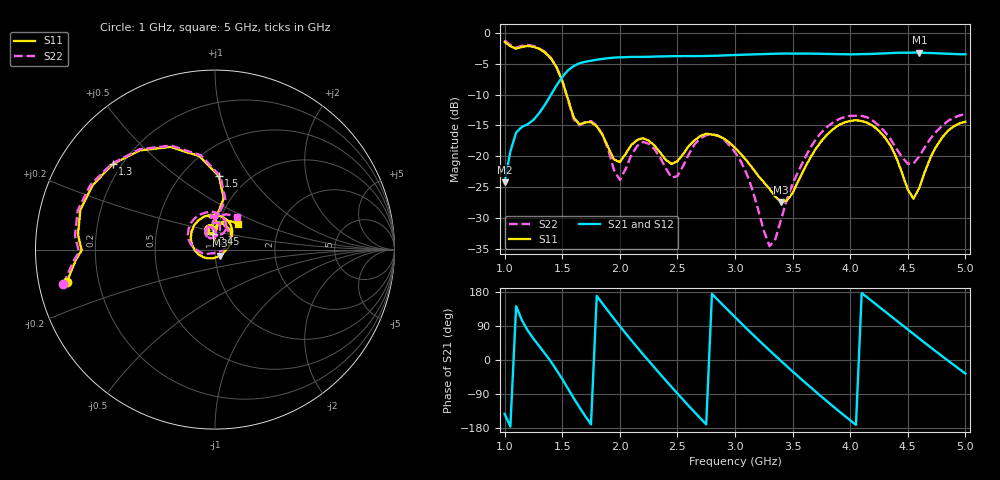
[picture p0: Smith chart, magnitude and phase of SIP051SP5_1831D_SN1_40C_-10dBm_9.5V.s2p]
# GHz  S  dB  R  50
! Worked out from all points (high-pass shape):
!   81 points, 1 GHz to 5 GHz, reference 50 ohm
!   highest |S21| = -3.22 dB at 4.6 GHz (marker M1); lowest = -24.2 dB at 1 GHz (marker M2)
!   |S21| within 3 dB of the highest: 1.544 GHz to end of sweep
!   lowest |S11| = -27.4 dB at 3.4 GHz (marker M3), VSWR 1.09, Z = 52.5 - j3.57 ohm
!   |S11| at or under -10 dB: 1.538 GHz to end of sweep
!   |S22| runs from -34.6 to -1.2 dB; largest |S21 - S12| = 0.0029
!   S11 on the Smith chart (normalised r, x): 1 GHz: 0.09, -0.11; 1.3 GHz: 0.17, +0.35; 1.5 GHz: 0.74, +0.73; 2.45 GHz: 0.96, +0.17; 5 GHz: 1.24, +0.36
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1  -1.48 -167.8  -24.22 -142.1  -24.22 -142.5  -1.25 -167.1
1.1  -2.58 -179.7  -16.16 141.9  -16.14 141.7  -2.41 -179.0
1.3  -2.58 140.2  -13.02 36.8  -13.04 36.7  -2.52 140.3
1.5  -7.75 87.0  -7.17 -50.1  -7.16 -50.2  -7.78 85.6
1.6  -13.72 85.2  -5.37 -100.7  -5.37 -100.7  -14.01 83.6
1.7  -14.52 100.3  -4.69 -148.0  -4.70 -148.0  -14.46 101.3
1.85  -16.54 85.6  -4.23 148.7  -4.23 148.7  -16.51 79.5
2  -20.95 108.9  -3.98 89.5  -3.98 89.6  -23.82 106.9
2.2  -17.07 104.2  -3.91 15.6  -3.91 15.7  -17.67 108.3
2.35  -19.39 89.0  -3.83 -37.1  -3.83 -37.1  -20.21 87.2
2.45  -21.24 97.5  -3.79 -71.5  -3.80 -71.5  -23.48 99.9
2.6  -18.29 106.8  -3.77 -121.8  -3.78 -121.6  -19.63 117.4
2.75  -16.34 83.9  -3.76 -169.9  -3.75 -169.9  -16.57 94.3
3  -18.63 38.6  -3.60 113.1  -3.59 113.1  -19.33 38.9
3.3  -25.29 -13.9  -3.41 25.4  -3.42 25.3  -34.55 -70.1
3.4  -27.38 -52.5  -3.38 -2.7  -3.38 -2.7  -30.24 -136.7
3.7  -18.84 -179.3  -3.39 -83.6  -3.39 -83.6  -17.30 168.2
4.05  -14.15 96.6  -3.48 -171.3  -3.48 -171.2  -13.43 104.7
4.35  -18.27 39.7  -3.29 116.6  -3.30 116.6  -17.23 62.7
4.6  -25.08 89.0  -3.22 56.5  -3.22 56.6  -20.00 92.4
4.8  -16.93 83.0  -3.36 9.6  -3.37 9.6  -15.03 87.3
5  -14.41 47.7  -3.48 -35.8  -3.49 -35.8  -13.16 55.9
